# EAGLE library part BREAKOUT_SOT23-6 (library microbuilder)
IC Breakout SOT23-6
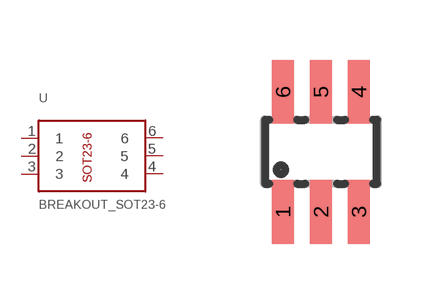
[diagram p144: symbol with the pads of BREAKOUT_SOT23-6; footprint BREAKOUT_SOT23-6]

Designator prefix U

## BREAKOUT_SOT23-6  [BREAKOUT_SOT23-6]
1  1
2  2
3  3
4  4
5  5
6  6

## Footprint BREAKOUT_SOT23-6 (pad centres in mm)
smd 0.55 x 1.6: 1 -0.95,-1.5; 2 0,-1.5; 3 0.95,-1.5; 4 0.95,1.5; 5 0,1.5; 6 -0.95,1.5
